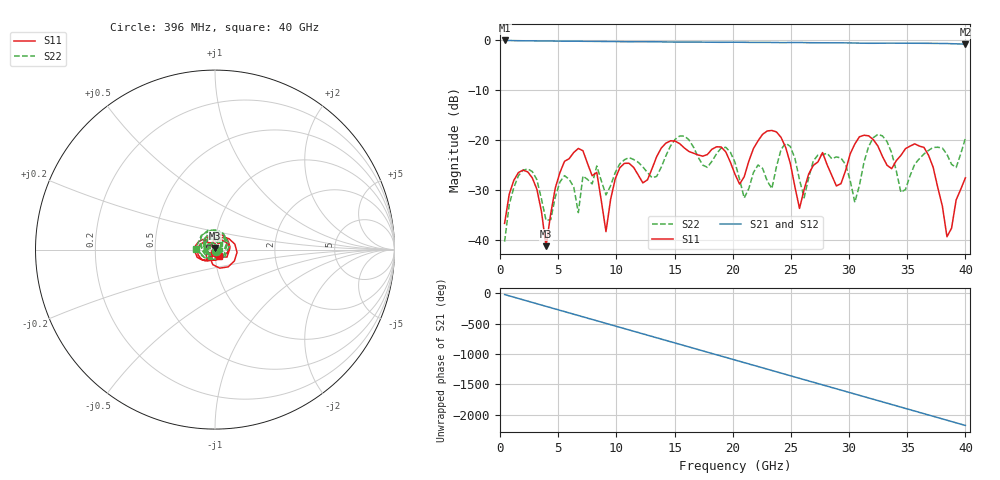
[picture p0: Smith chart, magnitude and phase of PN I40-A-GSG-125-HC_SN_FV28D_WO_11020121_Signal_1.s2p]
!  2-Port S-parameters as saved by WinCal
!VAR DATE=11-15-2012  13:25:18
!VAR OPNAME=Lynh Bui
# Hz S RI R 50.00
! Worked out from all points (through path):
!   101 points, 396 MHz to 40 GHz, reference 50 ohm
!   highest |S21| = -0.05 dB at 396 MHz (marker M1); lowest = -0.8 dB at 40 GHz (marker M2)
!   group delay of S21, straight-line fit = 151 ps
!   lowest |S11| = -41.2 dB at 3.96 GHz (marker M3), VSWR 1.02, Z = 49.8 + j0.851 ohm
!   |S11| at or under -10 dB: start of sweep to end of sweep
!   |S22| runs from -40.3 to -18.8 dB; largest |S21 - S12| = 0
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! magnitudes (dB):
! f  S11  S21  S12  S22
! 396 MHz  -36.6  -0.1  -0.1  -40.3
! 2.376 GHz  -26.3  -0.1  -0.1  -25.7
! 3.96 GHz  -41.2  -0.2  -0.2  -36.1
! 5.149 GHz  -26.5  -0.2  -0.2  -28.4
! 6.733 GHz  -21.6  -0.2  -0.2  -34.5
! 7.129 GHz  -22.1  -0.2  -0.2  -27.2
! 9.109 GHz  -38.3  -0.3  -0.3  -30.9
! 10.3 GHz  -25.5  -0.3  -0.3  -24.7
! 13.86 GHz  -21.6  -0.3  -0.3  -25.4
! 20.2 GHz  -26.8  -0.4  -0.4  -24.4
! 20.99 GHz  -27.3  -0.4  -0.4  -31.6
! 23.76 GHz  -18.3  -0.5  -0.5  -25.3
! 25.74 GHz  -33.6  -0.5  -0.5  -27.9
! 26.93 GHz  -25.0  -0.5  -0.5  -24.1
! 29.31 GHz  -28.7  -0.5  -0.5  -23.6
! 30.5 GHz  -20.8  -0.6  -0.6  -32.4
! 32.08 GHz  -19.9  -0.6  -0.6  -19.5
! 33.66 GHz  -25.7  -0.6  -0.6  -22.5
! 34.46 GHz  -23.0  -0.6  -0.6  -30.4
! 36.44 GHz  -21.4  -0.6  -0.6  -22.8
! 38.42 GHz  -39.3  -0.7  -0.7  -22.8
! 40 GHz  -27.5  -0.8  -0.8  -19.6
